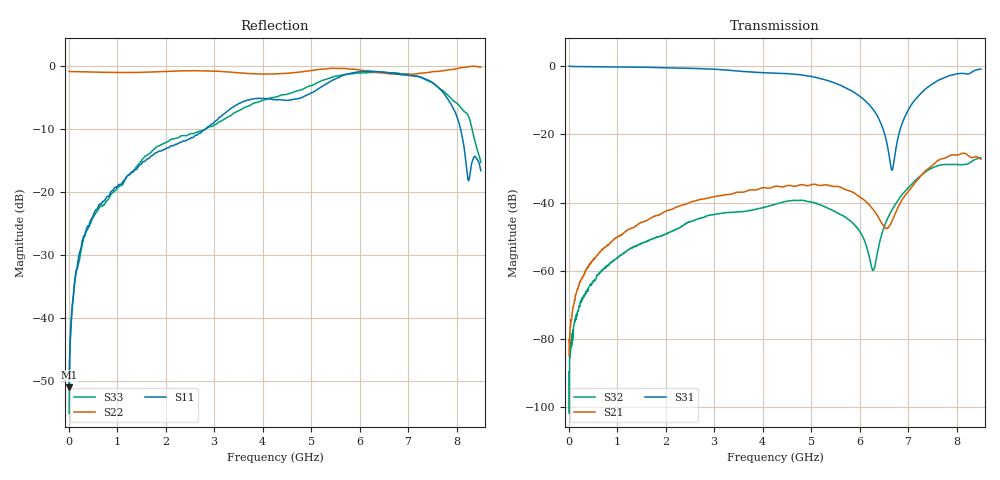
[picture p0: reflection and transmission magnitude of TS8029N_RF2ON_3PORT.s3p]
!Created with skrf (http://scikit-rf.org).
# GHz S RI R 50.0
!freq ReS11 ImS11 ReS12 ImS12 ReS13 ImS13
! ReS21 ImS21 ReS22 ImS22 ReS23 ImS23
! ReS31 ImS31 ReS32 ImS32 ReS33 ImS33
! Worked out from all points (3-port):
!   1601 points, 10 MHz to 8.5 GHz, reference 50 ohm
!   strongest paths, dB at 10 MHz, 2.132 GHz, 4.255 GHz, 6.378 GHz, 8.5 GHz:
!     S31: 0.0, -0.6, -2.1, -14.9, -0.9
!     S21: -84.8, -41.9, -35.2, -44.0, -27.3
!     S32: -89.6, -48.4, -40.5, -53.8, -26.8
!   lowest |S11| = -51.0 dB at 10 MHz (marker M1), VSWR 1.01, Z = 50 + j0.28 ohm
!   |S11| at or under -10 dB: start of sweep to 2.821 GHz; 8.082 GHz to end of sweep
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0.01  0.000231 0.0028  3.48e-05 6.15e-05  0.9948 -0.00815
      3e-05 4.93e-05  -0.9058 0.00332  3.69e-05 1.99e-05
      0.9947 -0.00826  3.27e-05 -5.67e-06  0.00155 0.000811
0.1479625  0.00868 -0.0216  0.000107 0.00044  0.9809 -0.0567
           6.35e-05 0.000439  -0.9018 0.0353  4.79e-05 -0.000214
           0.9808 -0.0569  4.89e-05 -0.000211  0.00623 -0.021
0.6149125  -0.00104 -0.0774  -0.000122 0.00177  0.9505 -0.2221
           -0.000121 0.00178  -0.8807 0.1525  -0.000518 -0.000713
           0.9506 -0.2219  -0.000526 -0.000728  -0.0127 -0.0726
4.255  -0.5406 0.0287  0.0088 0.015  -0.0774 -0.7838
       0.00879 0.0149  -0.319 0.8038  -0.000272 0.00944
       -0.0783 -0.7821  -0.00025 0.00943  -0.5648 -0.00678
5.692994  -0.5315 0.6626  0.0136 0.00761  -0.353 -0.3352
          0.0137 0.00762  -0.0136 0.9552  0.00452 0.00421
          -0.3531 -0.3352  0.00456 0.0042  -0.5683 0.6417
6.276681  -0.2211 0.8801  0.00702 0.00373  -0.2114 -0.0961
          0.00703 0.00371  0.0263 0.9028  -0.000234 0.000986
          -0.2116 -0.0962  -0.000211 0.000999  -0.379 0.8069
6.669344  0.048 0.8745  -0.00126 0.00524  -0.00115 -0.0298
          -0.00127 0.00524  0.1526 0.8502  -0.00742 0.00255
          -0.00123 -0.0297  -0.00741 0.00255  0.0565 0.8822
7.178744  0.4636 0.687  -0.00826 0.0191  0.2473 -0.237
          -0.00834 0.0191  0.3788 0.7819  -0.014 0.0171
          0.2478 -0.2371  -0.014 0.0171  0.5522 0.6186
8.022438  0.3791 0.000471  0.0214 0.0449  0.0096 -0.7693
          0.0215 0.045  0.5805 0.7605  0.0119 0.0341
          0.00968 -0.7703  0.0118 0.034  0.4519 0.2141
8.5  0.0848 0.1207  0.0248 0.0353  -0.2269 -0.8745
     0.0248 0.0353  0.5247 0.8263  0.0179 0.0419
     -0.2272 -0.8742  0.0179 0.0419  0.1709 -0.0126
